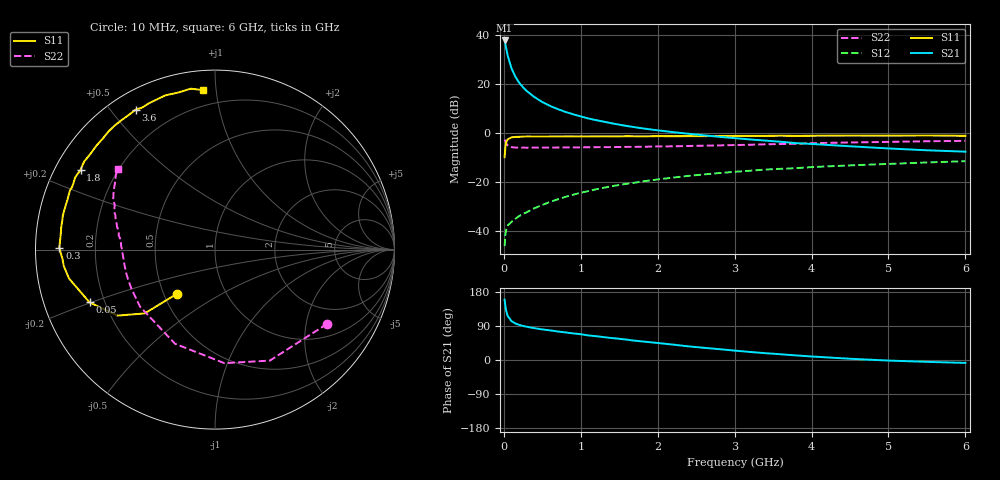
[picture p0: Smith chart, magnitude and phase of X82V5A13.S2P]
! SIEMENS Small Signal Semiconductors
! BFP136W
! Si NPN RF Bipolar Junction Transistor in SOT343
! VCE = 2.5 V  IC = 130 mA
! Common Emitter S-Parameters:  September  1994
# GHz  S  MA  R  50
!  f  S11  S21  S12  S22
! GHz  MAG  ANG  MAG  ANG  MAG  ANG  MAG  ANG
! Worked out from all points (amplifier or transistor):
!   40 points, 10 MHz to 6 GHz, reference 50 ohm
!   highest |S21| = 37.9 dB at 10 MHz (marker M1)
!   |S21| within 3 dB of that: start of sweep to 29.41 MHz
!   unconditionally stable (mu >= 1): 455.7 MHz to 2.929 GHz
!   at 200 MHz: K = 0.75, MSG = 27.2 dB, |S12| = -33.7 dB
!   at 1.5 GHz: K = 1.11, MAG = 10.3 dB, |S12| = -21.1 dB
!   at 6 GHz: K = 0.98, MSG = 1.9 dB, |S12| = -11.3 dB
!   S11 on the Smith chart (normalised r, x): 10 MHz: 0.58, -0.32; 50 MHz: 0.14, -0.20; 300 MHz: 0.07, +0.01; 1.8 GHz: 0.07, +0.27; 3.6 GHz: 0.07, +0.58; 6 GHz: 0.11, +0.92
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0.01  0.3268 -130.8  78.75 159.0  0.005 65.2  0.7496 -33.5
0.02  0.5293 -137.8  66.55 141.8  0.0084 56.2  0.6898 -63.7
0.03  0.6559 -145.9  55.13 130.0  0.0107 47.3  0.6348 -85.3
0.05  0.7583 -157.2  38.72 116.3  0.0132 39.6  0.5699 -113.0
0.1  0.8293 -168.8  21.16 102.4  0.0157 38.1  0.5248 -142.8
0.15  0.8477 -173.9  14.36 96.3  0.0181 42.4  0.5141 -154.8
0.2  0.8513 -176.5  10.77 92.6  0.0207 44.8  0.5122 -161.1
0.25  0.8609 -179.0  8.691 89.8  0.0227 47.6  0.5118 -165.2
0.3  0.8674 179.3  7.263 87.7  0.0248 50.2  0.5111 -167.9
0.4  0.8641 176.0  5.475 83.9  0.0299 54.7  0.5118 -171.7
0.5  0.8639 173.5  4.363 80.8  0.0347 57.8  0.5126 -174.2
0.6  0.8657 171.7  3.64 78.2  0.0399 59.6  0.5137 -175.9
0.8  0.8684 167.5  2.749 72.8  0.0506 62.1  0.5163 -178.4
1.1  0.8676 161.5  2.012 64.9  0.0667 62.5  0.5209 178.7
1.4  0.8696 156.5  1.611 58.0  0.0834 61.8  0.5246 176.3
1.8  0.8707 149.3  1.268 49.0  0.1046 59.1  0.5329 173.1
2.2  0.8752 142.7  1.061 40.6  0.1253 55.8  0.545 170.0
3.2  0.8895 125.8  0.753 21.2  0.173 45.9  0.5864 161.1
3.6  0.8963 119.6  0.675 15.1  0.1895 42.0  0.6062 157.6
4.5  0.903 107.9  0.546 3.3  0.2226 33.3  0.6538 149.7
5.5  0.9066 98.6  0.452 -4.9  0.255 25.4  0.6907 143.1
6  0.8918 94.4  0.424 -7.7  0.2711 21.0  0.7047 140.2
